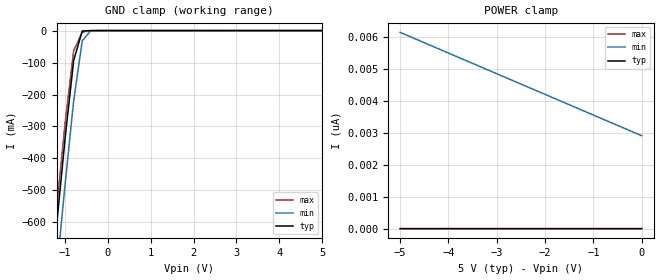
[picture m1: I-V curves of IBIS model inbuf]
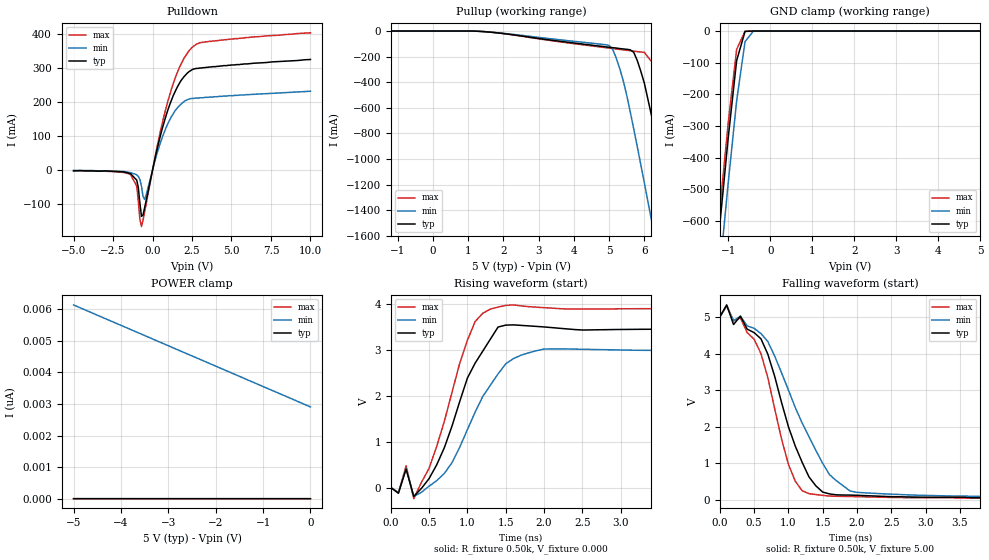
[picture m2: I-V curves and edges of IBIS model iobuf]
| IBIS file 4257k.ibs created by s2ibis2 version 1.0
| North Carolina State University Electronics Research Laboratory  1995
[IBIS ver]   2.1
[File name]   4257k.ibs
[File Rev]   0.1
[Date]   October 4, 2001
[Source]   IDT
[Notes]   1. Temp typ=25C, min=100C, max=0C 2. Ramp rates based on 500
   ohm load
[Copyright]   Copyright 2001, Integrated Device Technology, Inc.
|   Component IDT54/74FCT257T/AT/CT
[Component]   IDT54/74FCT257T/AT/CT
[Manufacturer]   Integrated Device Technology Inc.
[Package]
| Following package parameters are for D20-1(CDIP), P20-1(DPIP) packages
|[Package]
|| variable   typ   min   max
|R_pkg   40.00m   30.00m   50.00m
|L_pkg   7.00nH   4.00nH   10.00nH
|C_pkg   0.60pF   0.50pF   0.70pF
| Following package parameters are for SO20-6(EIAJ), SO20-2(SOIC) packages
|[Package]
|| variable   typ   min   max
|R_pkg   25.00m   20.00m   30.00m
|L_pkg   3.50nH   2.10nH   6.50nH
|C_pkg   0.40pF   0.35pF   0.60pF
| Following package parameters are for SO20-8(QSOP), SO20-7(SSOP) packages
| variable   typ   min   max
R_pkg   20.00m   15.00m   25.00m
L_pkg   3.00nH   2.00nH   4.00nH
C_pkg   0.30pF   0.26pF   0.34pF
[Pin]  signal_name   model_name   R_pin   L_pin   C_pin
1   S   inbuf
2   I0A   inbuf
3   I1A   inbuf
4   ZA   iobuf
5   I0B   inbuf
6   I1B   inbuf
7   ZB   iobuf
8   GND   GND
9   ZD   iobuf
10   I1D   inbuf
11   I0D   inbuf
12   ZC   iobuf
13   I1C   inbuf
14   I0C   inbuf
15   OEB   inbuf
16   VCC   POWER
| Models and submodels in the file (2): inbuf (Input), iobuf (I/O)
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| in   IN1   dummy_model
| oe   OE1   dummy_model
|   Model inbuf
[Model]   inbuf
Model_type   Input
Vinl =  0.800V
Vinh =  2.000V
C_comp   3.00pF   NA   NA
[Temperature Range]   25.00   100.00   0.000
[Voltage Range]   5.00V   4.50V   5.50V
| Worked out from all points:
|   GND clamp passes 1 mA (typ) near -0.55 V on its own axis
[GND_clamp]
| voltage   I(typ)   I(min)   I(max)
-5V       -6.185A    -6.347A    -6.076A
-1.4V     -895mA     -1.042A    -839mA
-1.2V     -612mA     -758mA     -559mA
-1V       -337mA     -481mA     -289mA
-800mV    -93.47mA   -220mA     -62.86mA
-600mV    -1.292mA   -32.12mA   -4.905mA
-400mV    -309nA     -162uA     -673uA
5V        467fA      3.231nA    197fA
[POWER_clamp]
| voltage   I(typ)   I(min)   I(max)
-5V       993fA      6.14nA     489fA
-4.5V     943fA      5.816nA    465fA
-4.2V     910fA      5.623nA    450fA
0V        467fA      2.908nA    224fA
|   Model iobuf
[Model]   iobuf
Model_type   I/O
Polarity   Non-Inverting
Enable   Active-High
Vinl =  0.800V
Vinh =  2.000V
C_comp   3.00pF   NA   NA
[Temperature Range]   25.00   100.00   0.000
[Voltage Range]   5.00V   4.50V   5.50V
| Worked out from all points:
|   slope of the pulldown table from 0 to 0.75 V, typ, clamps not added: 5.24 ohm
|   GND clamp passes 1 mA (typ) near -0.55 V on its own axis
|   rising waveform, R_fixture 0.50k, V_fixture 0.000: 20-80 % time 467ps typ, 551ps min, 407ps max; typ from 0 V to 3.46 V
|   falling waveform, R_fixture 0.50k, V_fixture 5.00: 20-80 % time 506ps typ, 708ps min, 395ps max; typ from 5 V to 0.046 V
[Pulldown]
| voltage   I(typ)   I(min)   I(max)
-5V       -2mA       -1mA       -1mA
-1.4V     -9.8mA     -7mA       -12mA
-1V       -29mA      -13.3mA    -46.5mA
-800mV    -96.13mA   -27mA      -143mA
-700mV    -135mA     -46.7mA    -165mA
-500mV    -110mA     -85.71mA   -122mA
300mV     63.4mA     50.88mA    70.83mA
900mV     166mA      129mA      190mA
1.5V      237mA      178mA      278mA
2.3V      288mA      208mA      349mA
3.1V      299mA      212mA      374mA
10V       324mA      231mA      402mA
[Pullup]
| voltage   I(typ)   I(min)   I(max)
-5V       0A         0A         0A
1.3V      -2.24mA    -2.654mA   -1.849mA
5V        -127mA     -113mA     -134mA
5.1V      -130mA     -143mA     -137mA
5.3V      -137mA     -292mA     -144mA
5.7V      -167mA     -767mA     -157mA
6V        -407mA     -1.187A    -167mA
6.4V      -905mA     -1.762A    -308mA
6.8V      -1.477A    -2.343A    -724mA
7.2V      -2.058A    -2.928A    -1.287A
7.6V      -2.644A    -3.515A    -1.867A
10V       -6.186A    -7.057A    -5.403A
[GND_clamp]
| voltage   I(typ)   I(min)   I(max)
-5V       -6.185A    -6.316A    -6.143A
-1.4V     -895mA     -1.038A    -848mA
-1.2V     -612mA     -756mA     -564mA
-1V       -337mA     -480mA     -290mA
-800mV    -93.47mA   -221mA     -57.95mA
-600mV    -1.292mA   -33.41mA   -728uA
-400mV    -309nA     -162uA     -18.34nA
5V        467fA      3.231nA    196fA
[POWER_clamp]
| voltage   I(typ)   I(min)   I(max)
-5V       994fA      6.14nA     485fA
-4.5V     942fA      5.816nA    459fA
-4.2V     909fA      5.623nA    443fA
0V        467fA      2.908nA    222fA
[Ramp]
| variable   typ   min   max
dV/dt_r   2.07/0.47n   1.80/0.55n   2.34/0.41n
dV/dt_f   2.97/0.51n   2.67/0.65n   3.28/0.43n
R_load = 0.50k
[Rising Waveform]
R_fixture = 0.50k
V_fixture = 0.000
| time   V(typ)   V(min)   V(max)
0s        0V         0V         0V
100ps     -124mV     -109mV     -120mV
200ps     402mV      423mV      475mV
300ps     -194mV     -194mV     -244mV
500ps     195mV      30.49mV    419mV
700ps     874mV      310mV      1.451V
1.1ns     2.715V     1.644V     3.623V
1.4ns     3.505V     2.482V     3.941V
2ns       3.507V     3.024V     3.928V
9.9ns     3.455V     2.999V     3.904V
[Falling Waveform]
R_fixture = 0.50k
V_fixture = 5.00
| time   V(typ)   V(min)   V(max)
0s        5V         5V         5V
100ps     5.326V     5.289V     5.318V
200ps     4.791V     4.896V     4.883V
300ps     5.019V     5.019V     4.974V
600ps     4.401V     4.545V     3.997V
1ns       2.005V     3.006V     981mV
1.3ns     634mV      1.732V     177mV
1.6ns     170mV      695mV      111mV
2ns       133mV      214mV      95mV
9.9ns     45.64mV    60.58mV    40.51mV
